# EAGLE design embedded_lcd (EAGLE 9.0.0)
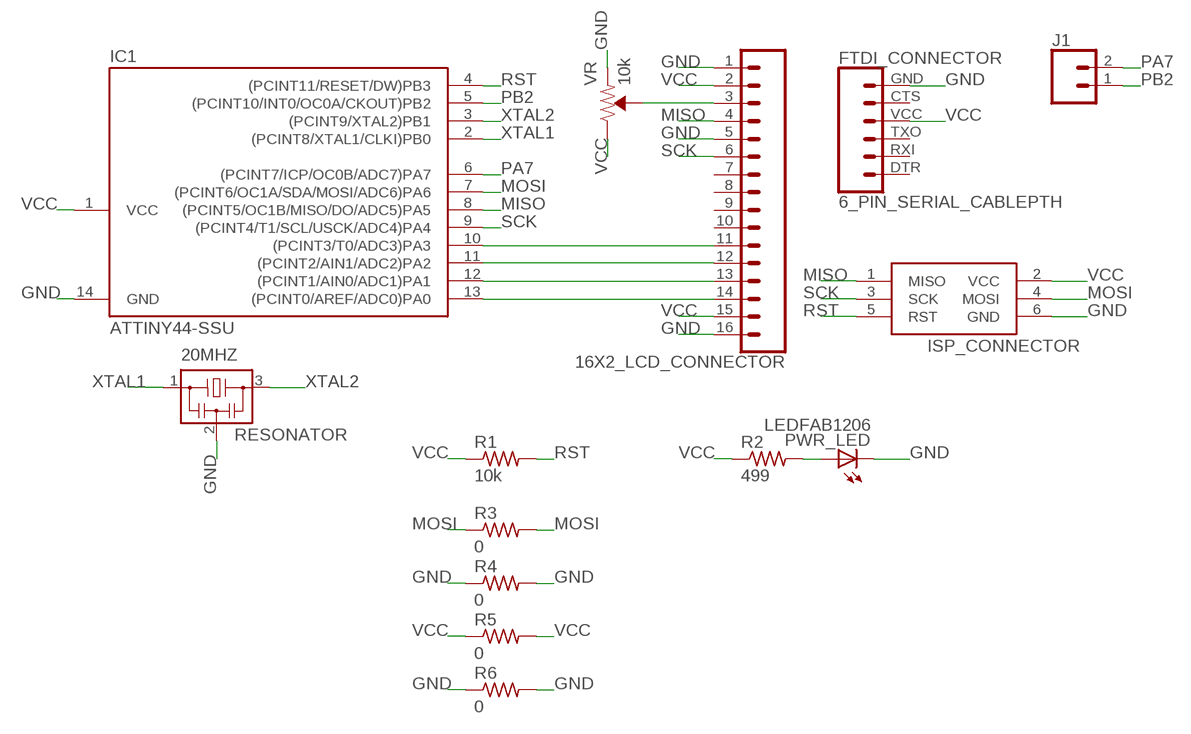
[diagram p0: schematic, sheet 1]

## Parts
16X2_LCD_CONNECTOR  CONN_16  [1X16]
20MHZ  RESONATOR  [EFOBM]
FTDI_CONNECTOR  6_PIN_SERIAL_CABLEPTH  [FTDI_BASIC]
IC1  ATTINY44-SSU  [SOIC14]
ISP_CONNECTOR  AVRISP-6  [AVRISP]
J1  CONN_02  [1X02]
PWR_LED  LEDFAB1206  [LED1206FAB]
R1  10k  RES-US1206FAB  [R1206FAB]
R2  499  RES-US1206FAB  [R1206FAB]
R3  0  RES-US1206FAB  [R1206FAB]
R4  0  RES-US1206FAB  [R1206FAB]
R5  0  RES-US1206FAB  [R1206FAB]
R6  0  RES-US1206FAB  [R1206FAB]
VR  10k  TRIMPOT-PTH-10MM-KNOB-1/2W-10%  [TRIMPOT-PTH-3386U]

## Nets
GND: 16X2_LCD_CONNECTOR.1 16X2_LCD_CONNECTOR.5 16X2_LCD_CONNECTOR.16 20MHZ.2 FTDI_CONNECTOR.GND IC1.14(GND) ISP_CONNECTOR.6(GND) PWR_LED.2(C) R4.1 R4.2 R6.1 R6.2 VR.1(CCW)
MISO: 16X2_LCD_CONNECTOR.4 IC1.8((PCINT5/OC1B/MISO/DO/ADC5)PA5) ISP_CONNECTOR.1(MISO)
MOSI: IC1.7((PCINT6/OC1A/SDA/MOSI/ADC6)PA6) ISP_CONNECTOR.4(MOSI) R3.1 R3.2
N$1: 16X2_LCD_CONNECTOR.14 IC1.13((PCINT0/AREF/ADC0)PA0)
N$2: 16X2_LCD_CONNECTOR.13 IC1.12((PCINT1/AIN0/ADC1)PA1)
N$3: 16X2_LCD_CONNECTOR.12 IC1.11((PCINT2/AIN1/ADC2)PA2)
N$4: 16X2_LCD_CONNECTOR.11 IC1.10((PCINT3/T0/ADC3)PA3)
N$5: PWR_LED.1(A) R2.2
N$8: 16X2_LCD_CONNECTOR.3 VR.2(WIPER)
PA7: IC1.6((PCINT7/ICP/OC0B/ADC7)PA7) J1.2
PB2: IC1.5((PCINT10/INT0/OC0A/CKOUT)PB2) J1.1
RST: IC1.4((PCINT11/RESET/DW)PB3) ISP_CONNECTOR.5(RST) R1.2
SCK: 16X2_LCD_CONNECTOR.6 IC1.9((PCINT4/T1/SCL/USCK/ADC4)PA4) ISP_CONNECTOR.3(SCK)
VCC: 16X2_LCD_CONNECTOR.2 16X2_LCD_CONNECTOR.15 FTDI_CONNECTOR.VCC IC1.1(VCC) ISP_CONNECTOR.2(VCC) R1.1 R2.1 R5.1 R5.2 VR.3(CW)
XTAL1: 20MHZ.1 IC1.2((PCINT8/XTAL1/CLKI)PB0)
XTAL2: 20MHZ.3 IC1.3((PCINT9/XTAL2)PB1)
Unconnected: 16X2_LCD_CONNECTOR.7 16X2_LCD_CONNECTOR.8 16X2_LCD_CONNECTOR.9 16X2_LCD_CONNECTOR.10 FTDI_CONNECTOR.CTS FTDI_CONNECTOR.DTR FTDI_CONNECTOR.RXI FTDI_CONNECTOR.TXO

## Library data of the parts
16X2_LCD_CONNECTOR = SparkFun-Connectors:CONN_16: Multi connection point. Often used as Generic Header-pin footprint for 0.1 inch spaced/style header connections On any of the 0.1 inch spaced packages, you can populate with these: Break Away Headers - Straight (PRT-00116) Break Away Male Headers - Right Angle (PRT-00553) Female Headers (PRT-00115)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
20MHZ = fab:RESONATOR
FTDI_CONNECTOR = SparkFun-Connectors:6_PIN_SERIAL_CABLE: 6-pin header connection for use with the "FTDI BASIC" pinout - CABLE SIDE. Also known as "Arduino Serial Program Header". This is used on a design to provide a 6-pin connection point for serial communication usually from a USB cable (D+/D-) to these headers (RX/TX). It also has the remaining pins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
IC1 = fab:ATTINY44
ISP_CONNECTOR = adafruit:AVRISP: AVR ISP HEADER Standard 6 pin header for AVR programming
J1 = SparkFun-Connectors:CONN_02: Multi connection point. Often used as Generic Header-pin footprint for 0.1 inch spaced/style header connections
PWR_LED = fab:LED: LED
R1-R6 = fab:RES-US: Resistor (US Symbol)
VR = SparkFun-Resistors:TRIMPOT: Trimming Potentiometer (Trimpot) Three-terminal potentiometers, with an adjustable wiper and two adjustable resistors. A pot can be used to create a configurable voltage divider, or as a variable resistor. "Trimpots" are a subset of potentiometers, usually intended for "set-and-forget"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; PROD_ID: RES-09730; SF_SKU: COM-09806

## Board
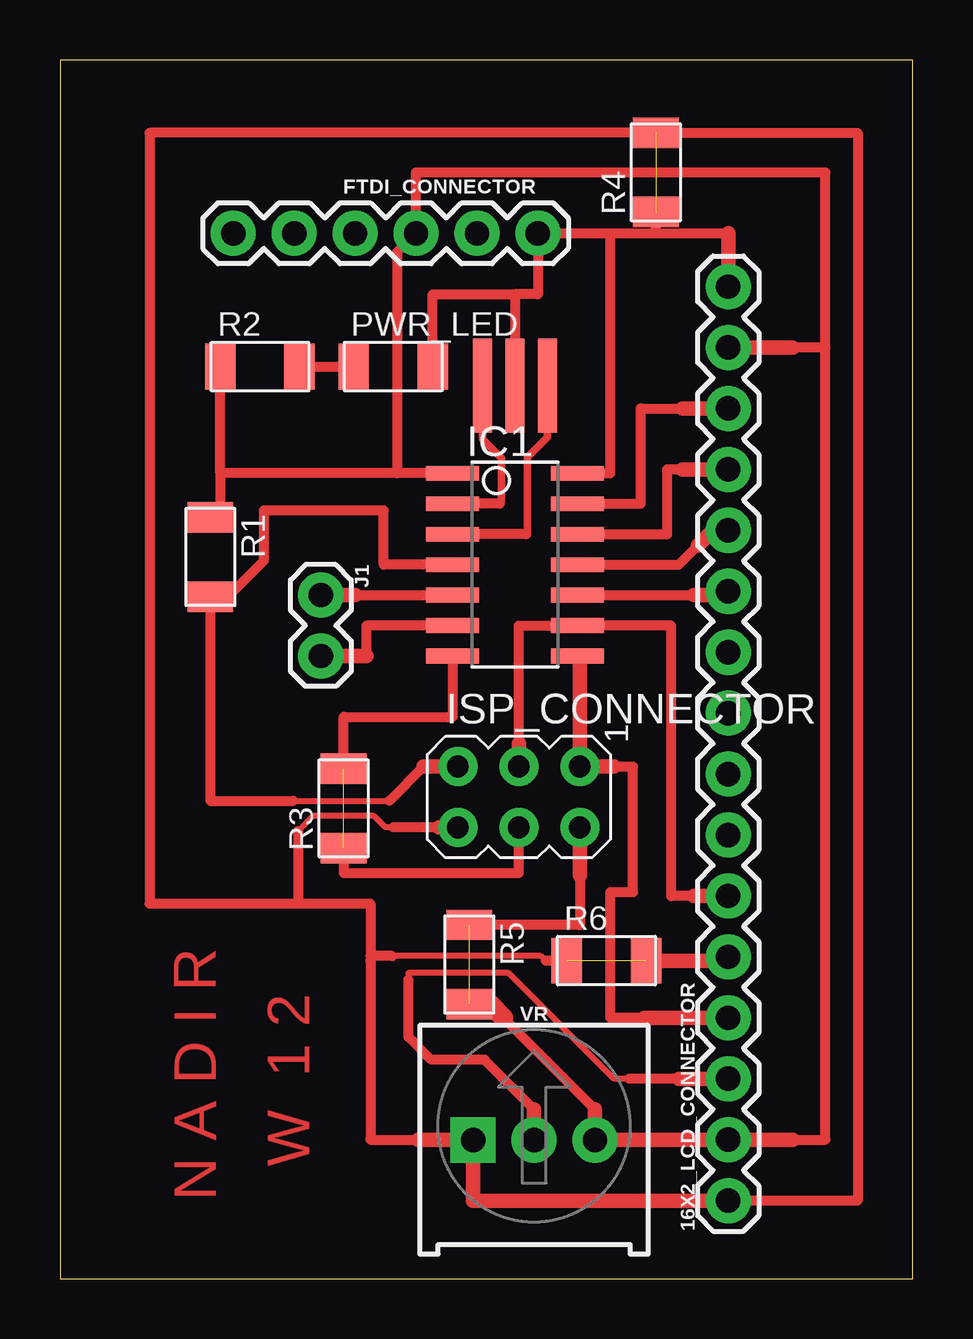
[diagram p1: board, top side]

Size 35.56 x 50.8 mm. Coordinates in mm from the lower left corner, seen from the top.
Outline: 0,0 35.56,0 35.56,50.8 0,50.8 0,0
Copper layers (1*16): Top 0.035mm / dielectric 1.5mm / Bottom 0.035mm
Design rules "default": minimum track width 6mil, minimum drill 0.35mm, track to track 6mil, track to pad 6mil, pad to pad 6mil, via to via 6mil, smd to smd 6mil, copper to edge 40mil, drill to drill 6mil, minimum pad ring 10mil, minimum via ring 8mil, stop-mask expansion 4mil, vias tented up to drill 0mil, thermal gap 10mil

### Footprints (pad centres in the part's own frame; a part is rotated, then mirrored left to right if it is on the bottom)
1X16 = drill 1.016 pad 1.88: 1 0,0; 2 2.54,0; 3 5.08,0; 4 7.62,0; 5 10.16,0; 6 12.7,0; 7 15.24,0; 8 17.78,0; 9 20.32,0; 10 22.86,0; 11 25.4,0; 12 27.94,0; 13 30.48,0; 14 33.02,0; 15 35.56,0; 16 38.1,0
EFOBM = smd 0.8 x 3.9: 1 -1.35,0; 2 0,0; 3 1.35,0
FTDI_BASIC = drill 1.016 pad 1.88: CTS 10.16,0; DTR 0,0; GND 12.7,0; RXI 2.54,0; TXO 5.08,0; VCC 7.62,0
SOIC14 = smd 0.61 x 2.21: 1 -3.81,-2.603; 2 -2.54,-2.603; 3 -1.27,-2.603; 4 0,-2.603; 5 1.27,-2.603; 6 2.54,-2.603; 7 3.81,-2.603; 8 3.81,2.603; 9 2.54,2.603; 10 1.27,2.603; 11 0,2.603; 12 -1.27,2.603; 13 -2.54,2.603; 14 -3.81,2.603
AVRISP = drill 0.9 pad 1.626: 1 -1.27,2.54; 2 1.27,2.54; 3 -1.27,0; 4 1.27,0; 5 -1.27,-2.54; 6 1.27,-2.54
1X02 = drill 1.016 pad 1.88: 1 0,0; 2 2.54,0
LED1206FAB = smd 1.27 x 1.905: 1 -1.651,0; 2 1.651,0
R1206FAB = smd 1.27 x 1.905: 1 -1.651,0; 2 1.651,0
TRIMPOT-PTH-3386U = drill 1.016 pad 1.88 square: 1 -2.54,-0.015 | drill 1.016 pad 1.88: 2 0,-0.015; 3 2.54,-0.015

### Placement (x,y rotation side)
16X2_LCD_CONNECTOR  27.86,3.25 90 top
20MHZ  18.97,37.23 0 top
FTDI_CONNECTOR  7.22,43.58 0 top
IC1  18.97,29.77 270 top
ISP_CONNECTOR  19.13,20.08 270 top
J1  10.87,28.5 270 top
PWR_LED  13.89,38.02 0 top
R1  6.27,30.08 270 top
R2  8.33,38.02 0 top
R3  11.83,19.61 90 top
R4  24.84,46.12 90 top
R5  17.07,13.1 270 top
R6  22.78,13.26 0 top
VR  19.76,5.79 0 top

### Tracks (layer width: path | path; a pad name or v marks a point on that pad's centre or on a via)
GND  (2 unrouted)
  Top 0.254: 13.89,18.81 13.57,18.81 13.1,19.29 10.56,19.29 9.92,18.65 | 20.24,13.26 20.04,13.45 13.85,13.45
  Top 0.406: 22.94,43.58 FTDI_CONNECTOR.GND 19.92,41.04 18.97,41.04 | PWR_LED.2 15.54,41.04 18.97,41.04 | 18.97,41.04 20MHZ.2 | IC1.14 22.94,33.58 22.94,43.58 | 15.8,18.81 13.89,18.81 | 9.92,18.65 9.92,15.64 | 22.94,43.58 24.84,43.58 | 24.84,43.58 R4.1 | 24.84,43.58 27.86,43.58 | 9.92,15.64 3.73,15.64 3.73,47.77 R4.2 33.26,47.77 33.26,3.25 16X2_LCD_CONNECTOR.1 | R6.1 20.24,13.26 | 9.92,15.64 12.94,15.64 12.94,13.45 | 14.92,5.79 12.94,5.79 12.94,13.26 12.94,13.45 | 13.85,13.45 12.94,13.45
  Top 0.61: 16X2_LCD_CONNECTOR.1 17.22,3.25 VR.1 17.22,5.79 14.92,5.79 | ISP_CONNECTOR.6 15.8,18.81 | 27.86,43.58 16X2_LCD_CONNECTOR.16 | R6.2 27.86,13.26 16X2_LCD_CONNECTOR.5
MISO
  Top 0.406: 23.1,21.35 23.89,21.35 23.89,16.11 22.94,16.11 22.94,10.87 24.37,10.87
  Top 0.61: IC1.8 21.67,25.96 ISP_CONNECTOR.1 23.1,21.35 | 16X2_LCD_CONNECTOR.4 24.37,10.87
MOSI  (1 unrouted)
  Top 0.406: R3.2 11.83,23.42 16.37,23.42 IC1.7 | R3.1 11.83,16.91 19.13,16.91 ISP_CONNECTOR.4
N$1
  Top 0.406: IC1.13 24.21,32.31 24.21,36.27 25.96,36.27
  Top 0.61: 25.96,36.27 16X2_LCD_CONNECTOR.14
N$2
  Top 0.406: IC1.12 25.32,31.04 25.32,33.73 25.96,33.73
  Top 0.61: 16X2_LCD_CONNECTOR.13 25.96,33.73
N$3
  Top 0.406: IC1.11 25.8,29.77 26.59,30.56
  Top 0.61: 26.59,30.56 27.23,31.19 16X2_LCD_CONNECTOR.12
N$4
  Top 0.406: IC1.10 26.43,28.5 | 16X2_LCD_CONNECTOR.11 27.7,28.5
  Top 0.61: 27.7,28.5 26.43,28.5
N$5
  Top 0.406: R2.2 PWR_LED.1
N$8
  Top 0.254: 23.73,8.33 23.1,8.33 18.69,12.74 14.53,12.74 14.53,12.46
  Top 0.406: 25.8,8.33 23.73,8.33 | 19.76,7.06 17.7,9.13 15.48,9.13 14.53,10.08 14.53,12.46
  Top 0.61: 16X2_LCD_CONNECTOR.3 25.8,8.33 | VR.2 19.76,7.06
PA7
  Top 0.406: IC1.6 12.78,27.23 12.78,25.96
  Top 0.61: J1.2 12.78,25.96
PB2
  Top 0.406: 12.3,28.5 IC1.5
  Top 0.61: J1.1 12.3,28.5
RST
  Top 0.254: 9.6,19.92 9.72,19.92 13.73,19.92
  Top 0.406: 15.16,21.35 13.73,19.92 | IC1.4 13.49,29.77 13.49,32.03 8.49,32.03 8.49,29.92 7.06,28.5 6.27,28.5 R1.2 6.27,19.92 9.72,19.92
  Top 0.61: ISP_CONNECTOR.5 15.16,21.35
SCK
  Top 0.406: 26.43,15.95 25.48,15.95 25.48,27.23 IC1.9 19.13,27.23 19.13,22.3
  Top 0.61: 16X2_LCD_CONNECTOR.6 26.43,15.95 | ISP_CONNECTOR.3 19.13,22.3
VCC  (1 unrouted)
  Top 0.406: IC1.1 14.05,33.58 | 14.05,33.58 14.05,42.78 FTDI_CONNECTOR.VCC 14.84,46.12 31.91,46.12 31.91,38.81 | 14.05,33.58 6.68,33.58 | 6.68,33.58 R2.1 | 6.68,33.58 6.68,31.73 R1.1 | 21.67,16.81 21.67,14.75 R5.1 | 22.3,7.06 18.49,10.87 | 30.56,5.79 31.91,5.79 31.91,38.81 | 31.91,38.81 30.56,38.81
  Top 0.61: 30.56,5.79 16X2_LCD_CONNECTOR.2 27.85,5.78 VR.3 22.3,7.06 | 30.56,38.81 16X2_LCD_CONNECTOR.15 | ISP_CONNECTOR.2 21.67,16.81
  Top 0.813: 18.49,10.87 17.92,11.45 R5.2
XTAL1
  Top 0.305: 20MHZ.1 17.62,35.01 18.41,34.21 18.41,32.38 18.34,32.31
  Top 0.406: 18.34,32.31 IC1.2 | 17.54,37.15 20MHZ.1
XTAL2
  Top 0.305: 20MHZ.3 20.32,35.08 19.49,34.25 19.49,31.07 19.45,31.04
  Top 0.406: 19.45,31.04 IC1.3

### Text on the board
Top: W 1 2 | N A D I R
